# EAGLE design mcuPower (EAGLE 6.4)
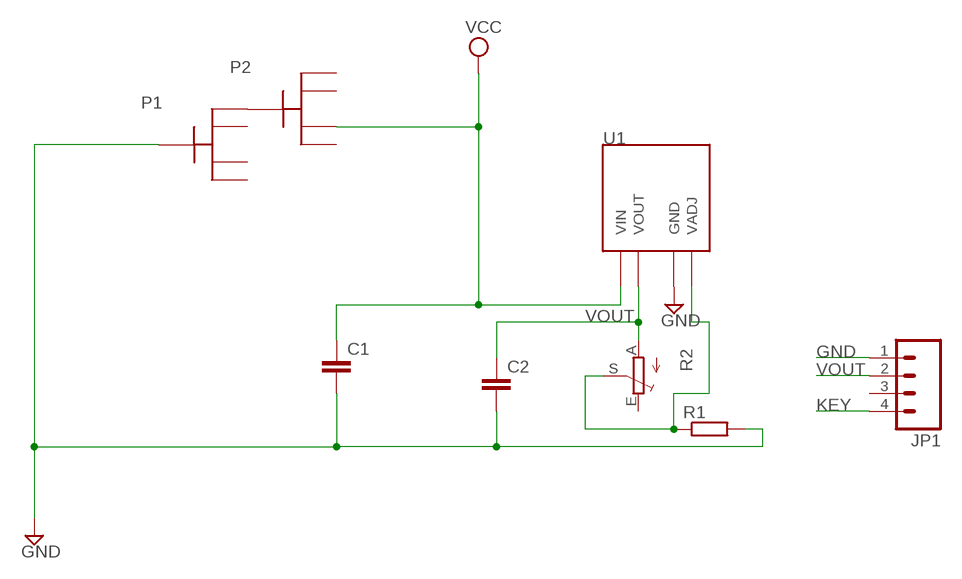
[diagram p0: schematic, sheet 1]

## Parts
C1  C-EUC0805  [C0805]
C2  C-EUC0805  [C0805]
JP1  M04PTH  [1X04]
P1  CR2032  [CR2032/2025]
P2  CR2032  [CR2032/2025]
R1  R-EU_R0805  [R0805]
R2  TRIM_EU-B25P  [B25P]
U1  PQ070XF01SZH  [TO220-4]

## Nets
GND: C1.2 C2.2 JP1.1 P1.GND R1.2 U1.GND
KEY: JP1.4
N$1: P1.VCC_1 P2.GND
N$2: R1.1 R2.S U1.VADJ
VCC: C1.1 P2.VCC_3 U1.VIN
VOUT: C2.1 JP1.2 R2.A U1.VOUT
Unconnected: JP1.3 P1.VCC_2 P1.VCC_3 P1.VCC_4 P2.VCC_1 P2.VCC_2 P2.VCC_4 R2.E

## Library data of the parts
C1 C2 = resistor:C-EU: CAPACITOR, European symbol
JP1 = SparkFun-Connectors:M04: Header 4 Standard 4-pin 0.1" header. Use with straight break away headers (SKU : PRT-00116), right angle break away headers (PRT-00553), swiss pins (PRT-00743), machine pins (PRT-00117), and female headers (PRT-00115). Molex polarized connector foot print use with SKU : PRT-08231 with associated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
P1 P2 = freddyLibr:CR2032: CR2032/2025 20mm 3V lithium coin cell Great for battery packup. Both SMT and THM holders. Note the THM package has the ground pads on both sides of the PCB so that the masks are the same - this reduces the cost
R1 = resistor:R-EU_: RESISTOR, European symbol
R2 = pot:TRIM_EU-: POTENTIOMETER
U1 = freddyLibr:PQ070XF01SZH: PQ070XF01SZH voltage regulator (TO220-4 package)

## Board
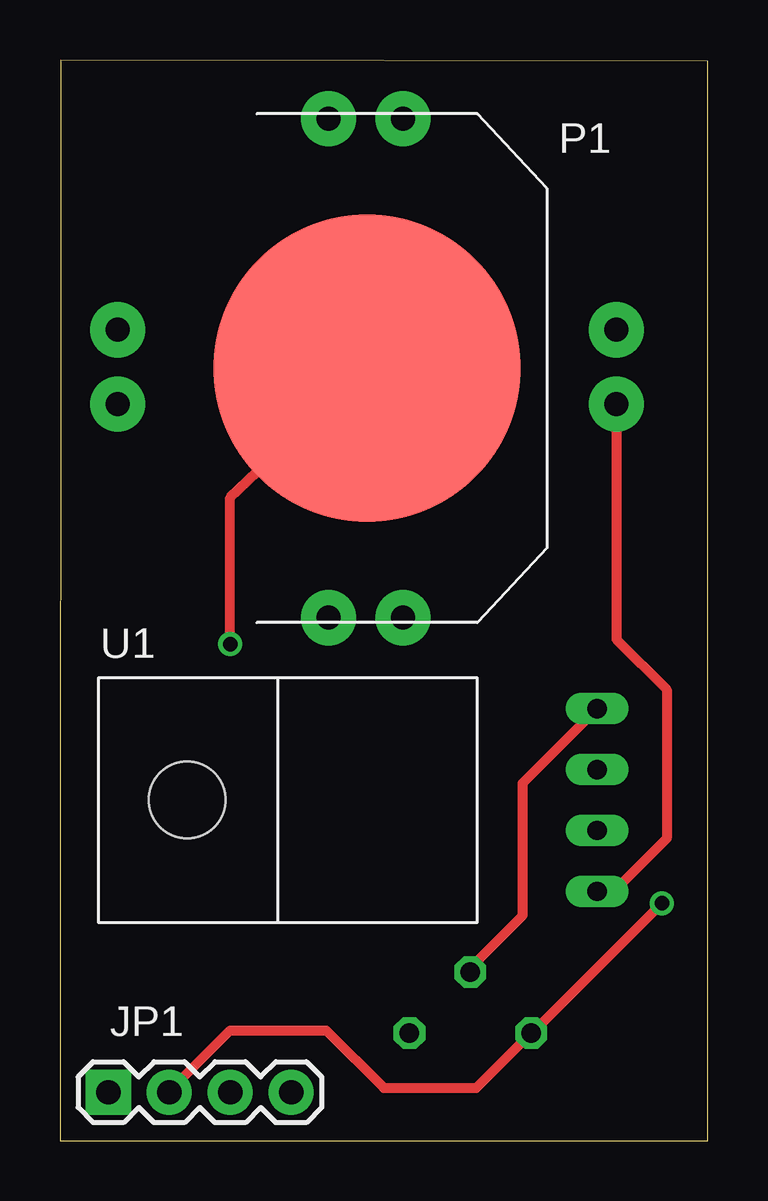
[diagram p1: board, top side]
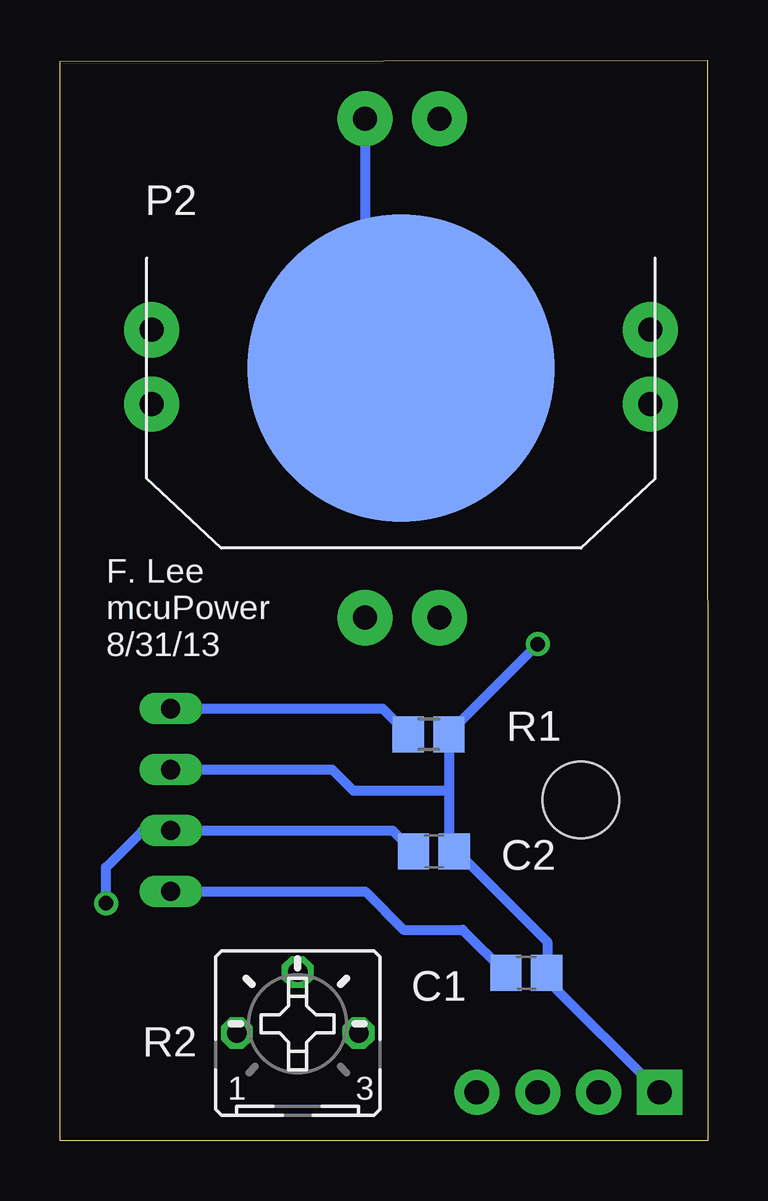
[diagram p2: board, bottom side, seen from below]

Size 27.02 x 45.05 mm. Coordinates in mm from the lower left corner, seen from the top.
Outline: 0,0 27.02,0 27.02,44.99 0.03,45.05 0,0
Copper layers (1*16): Top 0.035mm / dielectric 1.5mm / Bottom 0.035mm
Design rules "default *": minimum track width 10mil, minimum drill 20mil, track to track 8mil, track to pad 8mil, pad to pad 8mil, via to via 8mil, smd to smd 8mil, copper to edge 40mil, drill to drill 8mil, minimum pad ring 10mil, minimum via ring 8mil, stop-mask expansion 4mil, vias tented up to drill 0mil, thermal gap 10mil

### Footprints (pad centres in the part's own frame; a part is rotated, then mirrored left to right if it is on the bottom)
C0805 = smd 1.3 x 1.5: 1 -0.85,0; 2 0.85,0
1X04 = drill 1.016 pad 1.88 square: 1 0,0 | drill 1.016 pad 1.88: 2 2.54,0; 3 5.08,0; 4 7.62,0
CR2032/2025 = smd 12.8 x 12.8: GND 0,0 | drill 1 pad 2.3: VCC_1 -10.4,1.5; VCC_2 -10.4,-1.6; VCC_3 10.4,1.5; VCC_4 10.4,-1.6
R0805 = smd 1.3 x 1.5: 1 -0.85,0; 2 0.85,0
B25P = drill 0.813 octagon: A -2.54,0; E 2.54,0; S 0,2.54
TO220-4 = drill 0.8 long: GND 1.27,-13.3; VADJ 3.81,-13.3; VIN -3.81,-13.3; VOUT -1.27,-13.3 | hole 3.2: 0,3.8

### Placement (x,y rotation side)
C1  7.58,7 0 bottom
C2  11.43,12.06 0 bottom
JP1  2.02,2.02 0 top
P1  12.8,32.2 270 top
P2  12.8,32.2 180 bottom
R1  11.65,16.94 0 bottom
R2  17.11,4.49 0 bottom
U1  9.1,14.2 90 top

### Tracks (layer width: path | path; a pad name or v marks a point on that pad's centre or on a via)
GND  (via drill 0.6)
  Top 0.406: v7.1,20.7 7.1,26.8 P1.GND
  Bottom 0.406: JP1.1 6.73,6.73 C1.2 6.7,7.03 6.7,8.3 10.46,12.06 C2.2 10.8,12.28 10.8,14.6 | v7.1,20.7 10.8,17 R1.2 10.8,14.6 | U1.GND 15.67,15.47 14.8,14.6 10.8,14.6
N$1
  Bottom 0.406: P1.VCC_1 14.3,34 P2.GND
N$2
  Top 0.406: R2.S 17.11,7.21 19.3,9.4 19.3,14.91 U1.VADJ
  Bottom 0.406: U1.VADJ 13.57,18.01 R1.1
VCC
  Top 0.406: P2.VCC_3 23.2,20.9 25.3,18.8 25.3,12.6 23.1,10.4 U1.VIN
  Bottom 0.406: U1.VIN 14.29,10.39 12.7,8.8 10.23,8.8 C1.1
VOUT  (via drill 0.6)
  Top 0.406: v25.1,9.9 19.69,4.49 R2.A 17.36,2.2 13.5,2.2 11.1,4.6 7.1,4.6 4.56,2.06 JP1.2
  Bottom 0.406: C2.1 13.15,12.93 U1.VOUT 22.43,12.9 23.6,12.9 25.1,11.4 v25.1,9.9

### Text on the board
bPlace: F. Lee / mcuPower / 8/31/13

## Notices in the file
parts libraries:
SparkFun-Connectors: Licensing: CC v3.0 Share-Alike You are welcome to use this library for commercial purposes.
